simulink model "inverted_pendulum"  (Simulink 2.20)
settings: Solver=FixedStepDiscrete  StartTime=0.0  StopTime=5  FixedStep=0.01  RelTol=1e-3  AbsTol=1e-6
libraries: simulink x1

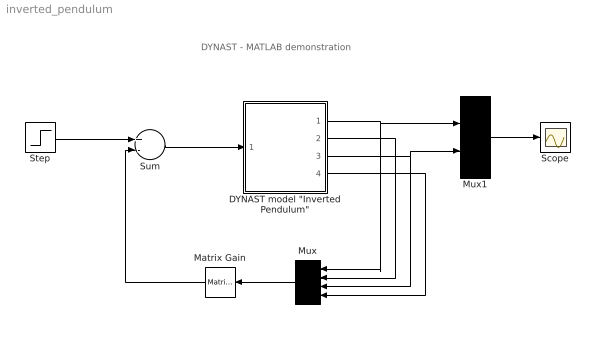
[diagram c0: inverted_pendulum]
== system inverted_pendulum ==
  note: DYNAST - MATLAB demonstration
  "DYNAST model \"Inverted Pendulum\"" : Subsystem
  Matrix Gain : simulink/Linear/Matrix Gain  Orientation=left  K="[-0.9384   -1.5565   18.1110    3.3499]"
  Mux : Mux  Orientation=left  Inputs=4
  Mux1 : Mux  Inputs=2
  Scope : Scope
  Step : Step  Time=0  Before=0  After=.2
  Sum : Sum  Inputs=+-
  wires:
  Sum/1 -> "DYNAST model \"Inverted Pendulum\""/1(u)
  Step/1 -> Sum/1
  Matrix Gain/1 -> Sum/2
  Mux/1 -> Matrix Gain/1
  Mux1/1 -> Scope/1
  "DYNAST model \"Inverted Pendulum\""/4("phidot ") -> Mux/4
  "DYNAST model \"Inverted Pendulum\""/3(phi) -> Mux1/2, Mux/3
  "DYNAST model \"Inverted Pendulum\""/2("xdot ") -> Mux/2
  "DYNAST model \"Inverted Pendulum\""/1(x) -> Mux1/1, Mux/1

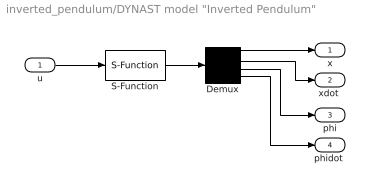
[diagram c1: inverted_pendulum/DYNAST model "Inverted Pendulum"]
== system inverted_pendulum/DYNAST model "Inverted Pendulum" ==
  u : Inport  Port=1  PortWidth=-1  SampleTime=-1
  Demux : Demux  Outputs=4
  S-Function : S-Function  FunctionName=dynPlantL  Parameters='%DYNAST%\examples\control\InvertedPendulum.prb',0.01  PortCounts=[]  SFunctionModules=''
  x : Outport  Port=1
  "xdot " : Outport  Port=2
  phi : Outport  Port=3
  "phidot " : Outport  Port=4
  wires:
  u/1 -> S-Function/1
  S-Function/1 -> Demux/1
  Demux/1 -> x/1
  Demux/2 -> "xdot "/1
  Demux/3 -> phi/1
  Demux/4 -> "phidot "/1
